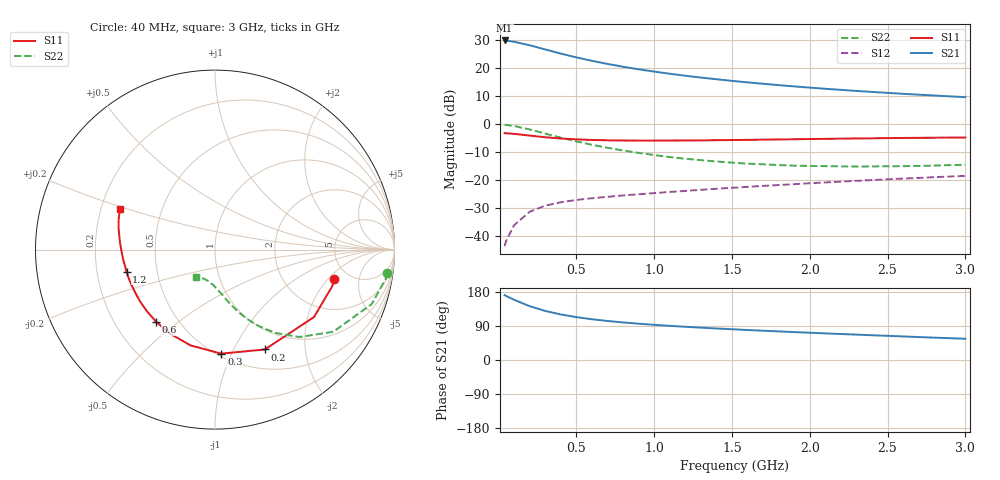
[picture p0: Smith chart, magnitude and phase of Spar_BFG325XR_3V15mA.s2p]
! Filename: 315BFG325XR.s2p
! Title: BFG325XR,RN20042071,Lot:TT3899C,B:Y13641,Sl.:1
! Bias: VCE=2.999V; IC=14.88mA;
! Company: NXP Semiconductors NL
! User: Q&R DSC-N
! Measure time: 29 Mar 2004 / 13:40:46
#  MHz  S  MA  R 50
! Freq  S11  S21  S12  S22  :
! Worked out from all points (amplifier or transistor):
!   32 points, 40 MHz to 3 GHz, reference 50 ohm
!   highest |S21| = 30.0 dB at 40 MHz (marker M1)
!   |S21| within 3 dB of that: start of sweep to 286.3 MHz
!   unconditionally stable (mu >= 1): 1.795 GHz to end of sweep
!   at 400 MHz: K = 0.42, MSG = 26.7 dB, |S12| = -28.0 dB
!   at 1.5 GHz: K = 0.95, MSG = 19.2 dB, |S12| = -22.9 dB
!   at 3 GHz: K = 1.05, MAG = 12.7 dB, |S12| = -18.6 dB
!   S11 on the Smith chart (normalised r, x): 40 MHz: 3.79, -2.38; 200 MHz: 0.74, -1.34; 300 MHz: 0.52, -0.92; 600 MHz: 0.38, -0.42; 1.2 GHz: 0.33, -0.11; 3 GHz: 0.28, +0.19
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40  0.6856 -14.0  31.51 171.1  0.006476 83.4  0.9699 -7.8
50  0.6838 -17.5  31.28 169.0  0.008008 81.7  0.965 -9.7
100  0.6675 -34.2  29.89 159.1  0.01529 74.4  0.9244 -19.2
200  0.6219 -63.5  25.87 142.2  0.02672 62.8  0.8025 -34.8
300  0.5807 -86.5  21.79 129.6  0.03441 55.3  0.676 -46.1
400  0.551 -104.2  18.36 120.2  0.03963 50.9  0.5706 -54.3
500  0.5316 -118.1  15.68 113.2  0.04363 48.6  0.4889 -60.4
600  0.519 -129.1  13.61 107.6  0.04679 47.4  0.4258 -65.2
700  0.5116 -138.1  11.97 103.0  0.04967 46.9  0.3758 -69.0
800  0.5076 -145.5  10.66 99.2  0.0525 46.9  0.3362 -72.3
900  0.5048 -151.8  9.603 95.8  0.05515 47.2  0.3046 -75.3
1000  0.5052 -157.2  8.722 92.8  0.05782 47.6  0.2788 -78.0
1100  0.5069 -161.8  7.984 90.1  0.06066 48.1  0.2564 -80.6
1200  0.508 -166.0  7.354 87.7  0.06336 48.6  0.239 -83.4
1300  0.5099 -169.8  6.818 85.4  0.0662 49.1  0.2253 -86.1
1400  0.5137 -173.2  6.362 83.2  0.06918 49.5  0.2137 -88.4
1600  0.5209 -179.0  5.592 79.1  0.07477 50.3  0.1952 -93.9
1800  0.5301 176.1  4.98 75.5  0.08077 51.0  0.184 -98.7
2100  0.5432 170.0  4.286 70.2  0.0898 51.4  0.1761 -106.2
2300  0.552 166.7  3.926 67.0  0.09617 51.6  0.1733 -110.7
2600  0.5633 162.2  3.484 62.2  0.1055 51.6  0.1759 -116.8
3000  0.5738 157.0  3.039 56.0  0.1178 50.7  0.1862 -123.8
